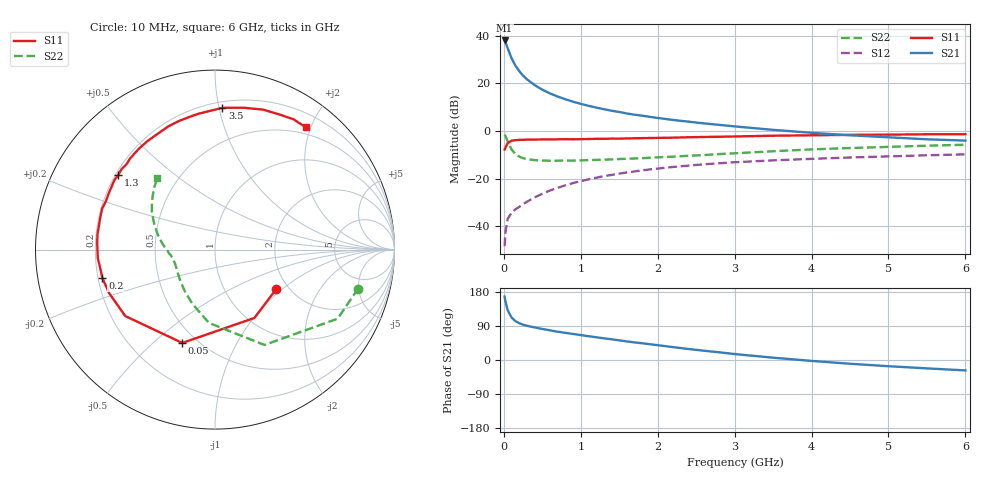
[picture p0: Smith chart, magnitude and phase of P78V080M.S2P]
! SIEMENS Small Signal Semiconductors
! BFP196
! Si NPN RF Bipolar Junction Transistor in SOT143
! VCE = 8 V  IC = 80 mA
! Common Emitter S-Parameters:  May  1996
# GHz  S  MA  R  50
!  f  S11  S21  S12  S22
! GHz  MAG  ANG  MAG  ANG  MAG  ANG  MAG  ANG
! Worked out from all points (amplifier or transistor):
!   36 points, 10 MHz to 6 GHz, reference 50 ohm
!   highest |S21| = 38.0 dB at 10 MHz (marker M1)
!   |S21| within 3 dB of that: start of sweep to 47.07 MHz
!   unconditionally stable (mu >= 1): 428.6 MHz to 4.837 GHz
!   at 250 MHz: K = 0.87, MSG = 27.0 dB, |S12| = -30.8 dB
!   at 1.4 GHz: K = 1.09, MAG = 11.7 dB, |S12| = -18.5 dB
!   at 6 GHz: K = 0.98, MSG = 2.9 dB, |S12| = -9.9 dB
!   S11 on the Smith chart (normalised r, x): 10 MHz: 1.74, -0.91; 50 MHz: 0.42, -0.62; 200 MHz: 0.22, -0.12; 1.3 GHz: 0.21, +0.33; 3.5 GHz: 0.24, +1.02; 6 GHz: 0.40, +1.92
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0.01  0.4061 -32.6  78.98 167.3  0.0038 78.9  0.8269 -15.2
0.02  0.4396 -60.0  72.87 155.4  0.0073 69.4  0.7842 -29.4
0.05  0.551 -109.3  54.33 131.3  0.0142 53.3  0.5984 -62.6
0.1  0.6221 -143.5  33.55 112.0  0.0191 47.2  0.4095 -94.8
0.15  0.6378 -157.7  23.49 102.7  0.0225 49.1  0.3268 -112.8
0.2  0.647 -165.8  17.98 97.1  0.0253 53.4  0.2885 -125.1
0.25  0.6489 -172.1  14.41 93.2  0.0289 54.9  0.2673 -134.2
0.3  0.6546 -175.8  12.09 90.4  0.0325 57.5  0.256 -140.2
0.4  0.6571 177.1  9.154 85.9  0.0402 60.7  0.2432 -149.3
0.5  0.6604 172.7  7.323 82.0  0.0477 62.2  0.2383 -155.1
0.6  0.6604 168.0  6.111 78.3  0.056 62.8  0.236 -159.0
0.7  0.6645 163.6  5.255 74.6  0.0636 62.6  0.2365 -162.2
0.9  0.6649 156.0  4.088 68.7  0.0804 61.7  0.238 -166.8
1.1  0.6739 148.9  3.358 62.8  0.096 60.2  0.2434 -170.0
1.3  0.6812 142.2  2.851 57.2  0.1122 57.4  0.2489 -172.9
1.7  0.6987 129.8  2.183 46.4  0.1409 52.2  0.2632 -178.3
2.2  0.7197 116.4  1.693 34.0  0.1748 44.7  0.2872 175.3
2.8  0.7523 101.1  1.336 20.3  0.209 35.8  0.3258 166.1
3.5  0.7911 87.0  1.05 6.1  0.2402 25.9  0.3733 155.9
4.5  0.8247 71.0  0.807 -9.9  0.276 14.0  0.4364 143.7
5.5  0.8478 58.9  0.665 -22.1  0.3073 3.4  0.4879 133.6
6  0.8486 53.4  0.625 -27.5  0.3215 -2.2  0.512 128.8
